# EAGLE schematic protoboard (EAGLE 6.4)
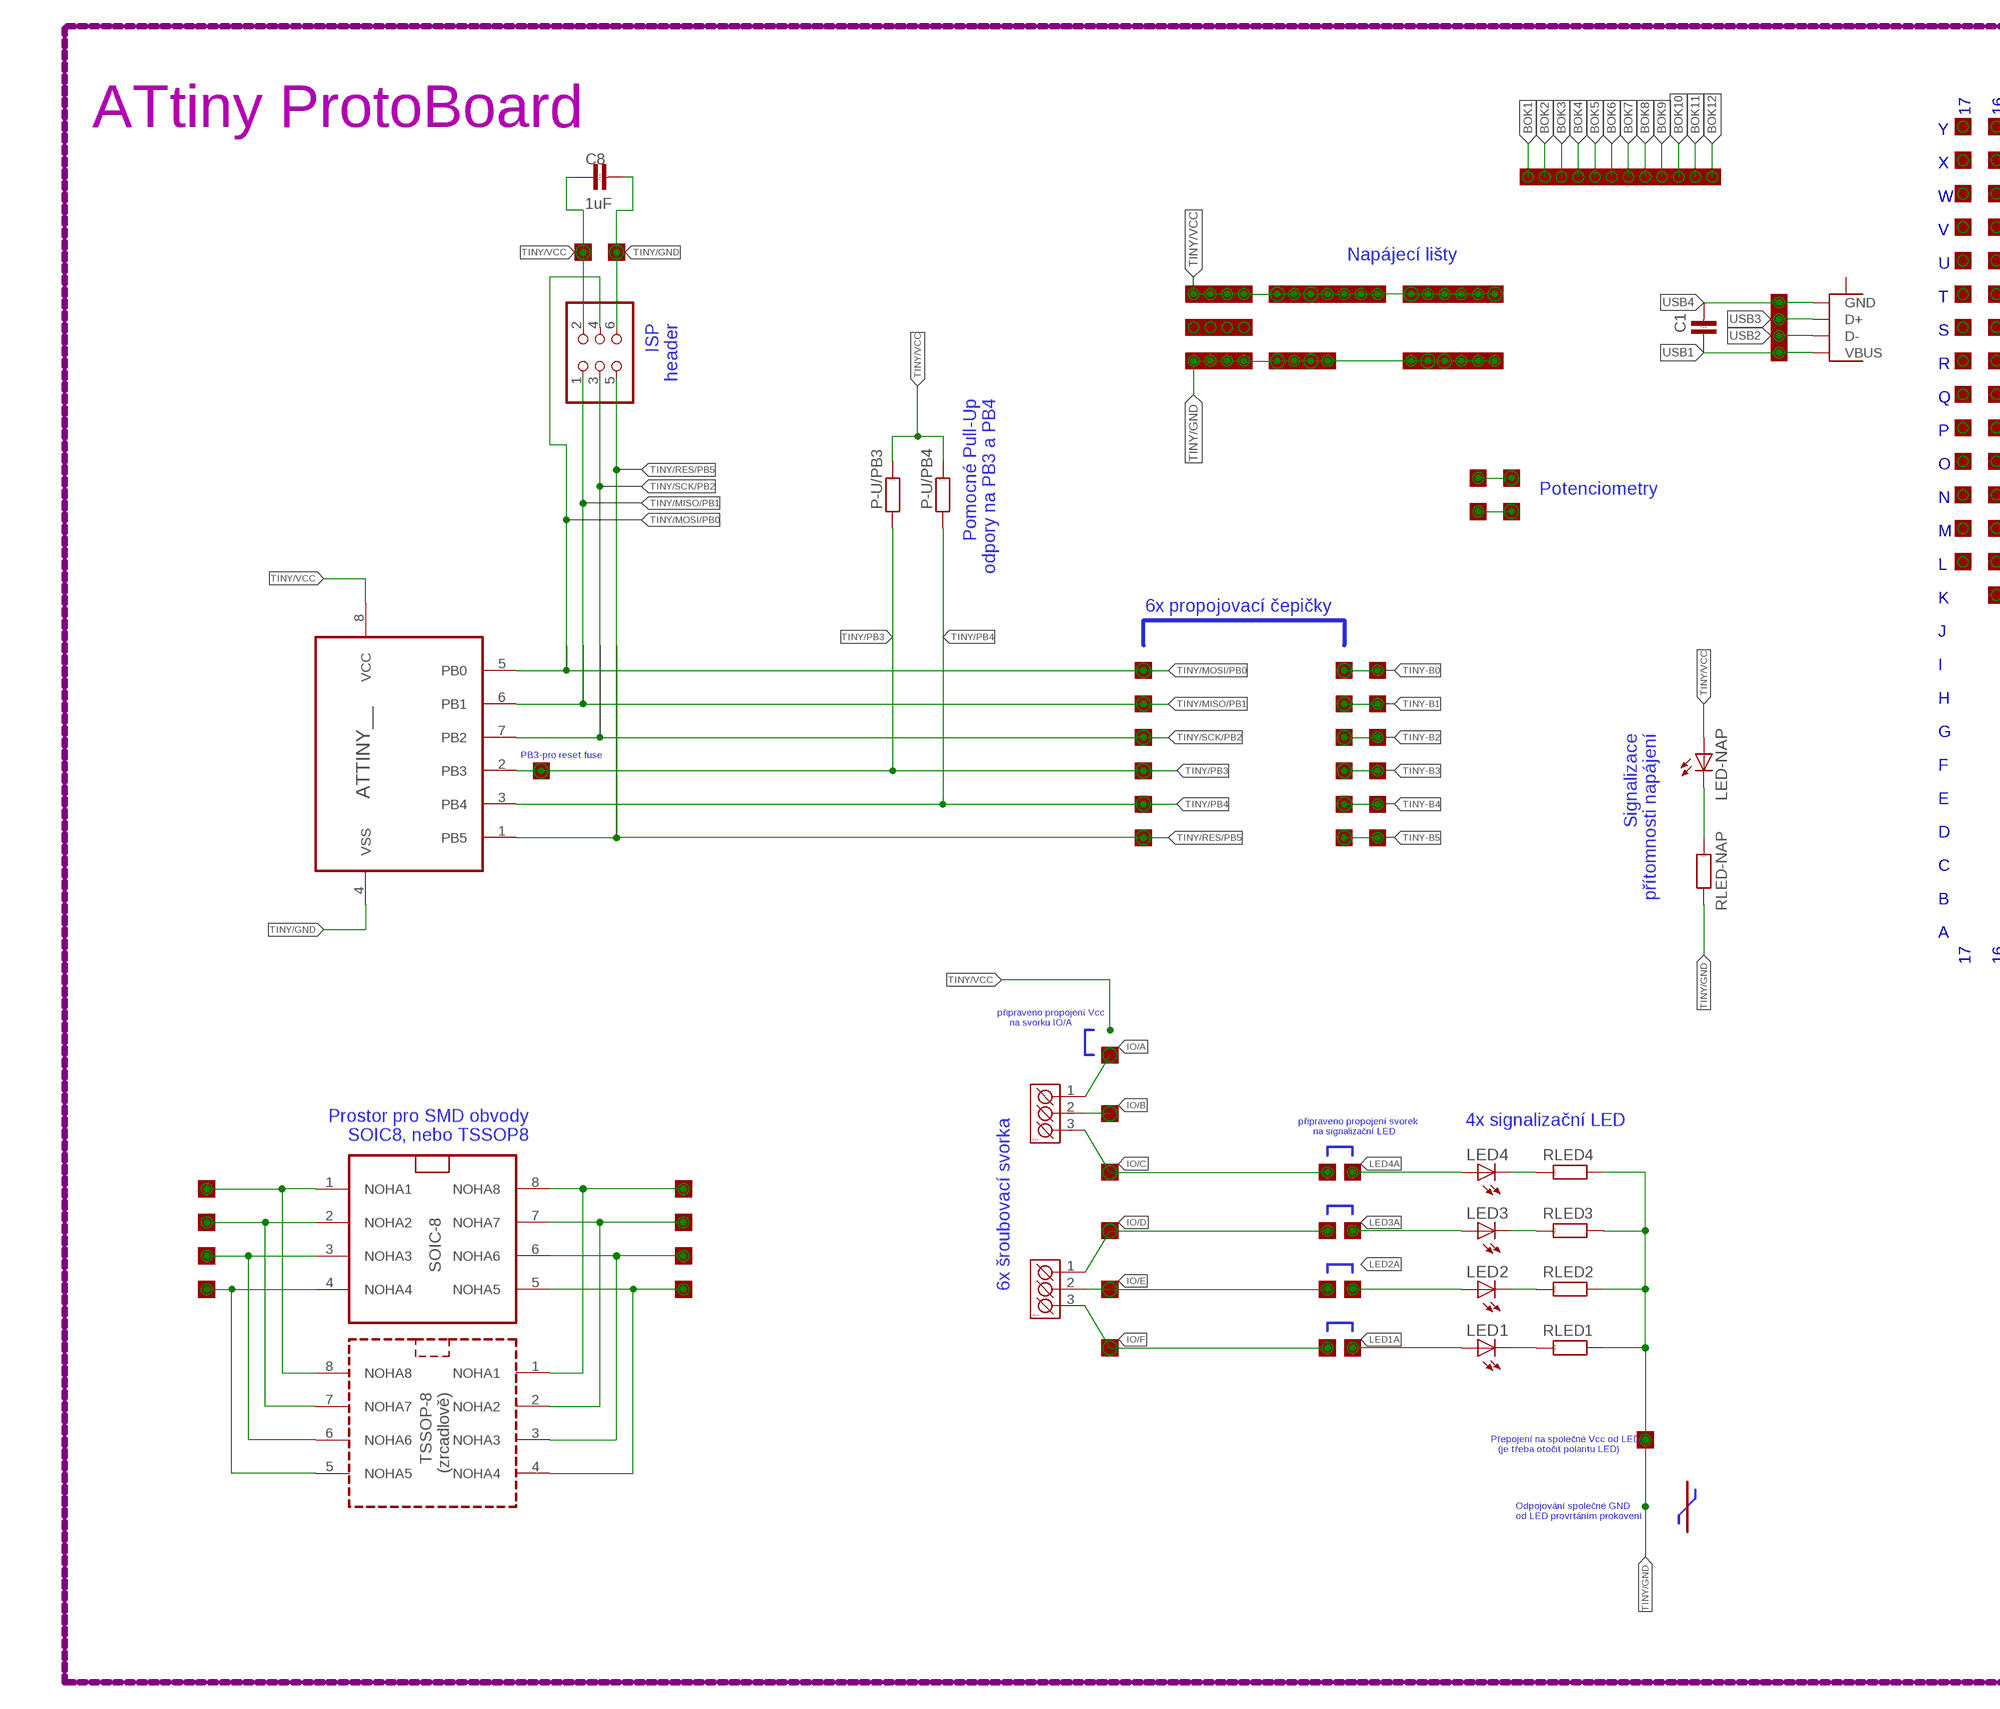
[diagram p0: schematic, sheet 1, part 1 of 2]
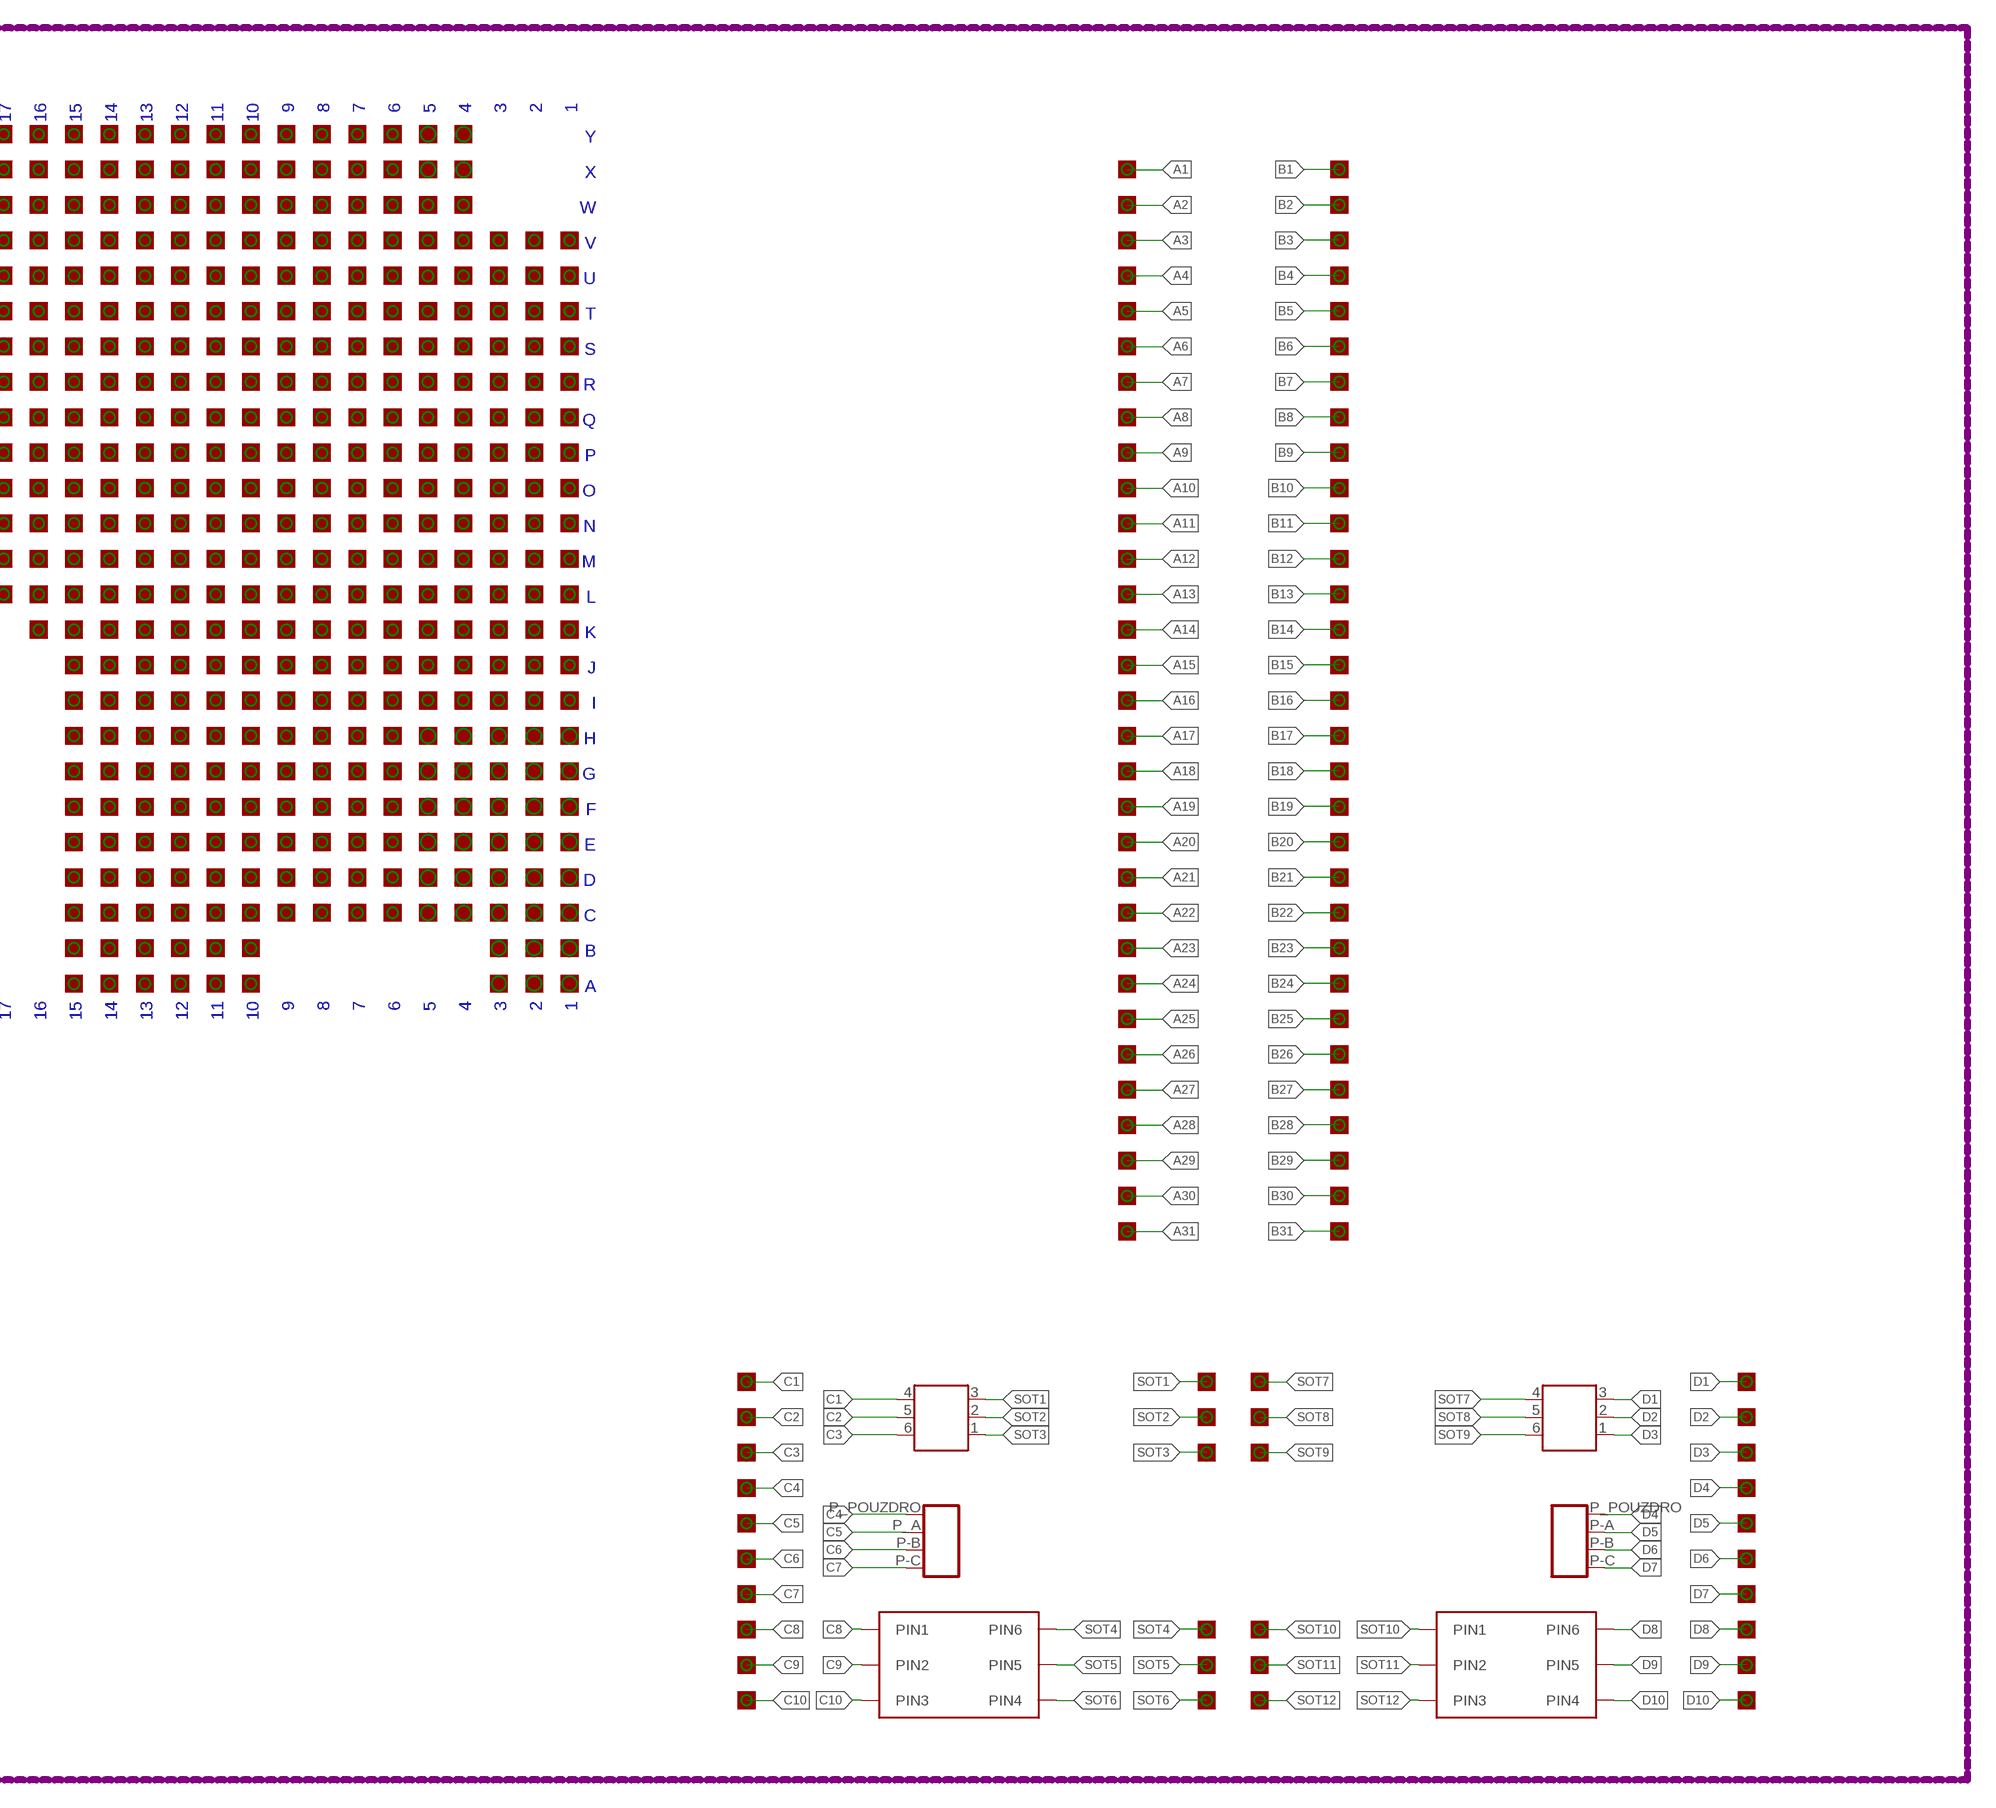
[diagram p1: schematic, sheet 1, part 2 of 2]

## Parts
ARK-A  PINHD-1X1  [1X01]
ARK-B  PINHD-1X1  [1X01]
ARK-C  PINHD-1X1  [1X01]
ARK-D  PINHD-1X1  [1X01]
ARK-E  PINHD-1X1  [1X01]
ARK-F  PINHD-1X1  [1X01]
ATTINY  ATTINY__  ATTINY13  [SOIC127P600X175-8N]
C1  C-KERAMIK_SMD_0805  [0805]
C8  1uF  C-KERAMIK_SMD_0805  [0805]
EMPTY1  SOIC-NIC  [SOIC127P600X175-8N]
EMPTY2  TSSOP-NIC  [TSSOP8]
IC1  AD8519KS  [SC70-5]
IC2  AD8519RJ  [SOT23-5]
J-A1  PINHD-1X1  [1X01]
J-A2  PINHD-1X1  [1X01]
J-A3  PINHD-1X1  [1X01]
J-A10  PINHD-1X1  [1X01]
J-A11  PINHD-1X1  [1X01]
J-A12  PINHD-1X1  [1X01]
J-A13  PINHD-1X1  [1X01]
J-A14  PINHD-1X1  [1X01]
J-A15  PINHD-1X1  [1X01]
J-B1  PINHD-1X1  [1X01]
J-B2  PINHD-1X1  [1X01]
J-B3  PINHD-1X1  [1X01]
J-B4  PINHD-1X1  [1X01]
J-B5  PINHD-1X1  [1X01]
J-B6  PINHD-1X1  [1X01]
J-B7  PINHD-1X1  [1X01]
J-B8  PINHD-1X1  [1X01]
J-B9  PINHD-1X1  [1X01]
J-B10  PINHD-1X1  [1X01]
J-B11  PINHD-1X1  [1X01]
J-B12  PINHD-1X1  [1X01]
J-B13  PINHD-1X1  [1X01]
J-B14  PINHD-1X1  [1X01]
J-B15  PINHD-1X1  [1X01]
J-C1  PINHD-1X1  [1X01]
J-C2  PINHD-1X1  [1X01]
J-C3  PINHD-1X1  [1X01]
J-C4  PINHD-1X1  [1X01]
J-C5  PINHD-1X1  [1X01]
J-C6  PINHD-1X1  [1X01]
J-C7  PINHD-1X1  [1X01]
J-C8  PINHD-1X1  [1X01]
J-C9  PINHD-1X1  [1X01]
J-C10  PINHD-1X1  [1X01]
J-C11  PINHD-1X1  [1X01]
J-C12  PINHD-1X1  [1X01]
J-C13  PINHD-1X1  [1X01]
J-C14  PINHD-1X1  [1X01]
J-C15  PINHD-1X1  [1X01]
J-D1  PINHD-1X1  [1X01]
J-D2  PINHD-1X1  [1X01]
J-D3  PINHD-1X1  [1X01]
J-D4  PINHD-1X1  [1X01]
J-D5  PINHD-1X1  [1X01]
J-D6  PINHD-1X1  [1X01]
J-D7  PINHD-1X1  [1X01]
J-D8  PINHD-1X1  [1X01]
J-D9  PINHD-1X1  [1X01]
J-D10  PINHD-1X1  [1X01]
J-D11  PINHD-1X1  [1X01]
J-D12  PINHD-1X1  [1X01]
J-D13  PINHD-1X1  [1X01]
J-D14  PINHD-1X1  [1X01]
J-D15  PINHD-1X1  [1X01]
J-E1  PINHD-1X1  [1X01]
J-E2  PINHD-1X1  [1X01]
J-E3  PINHD-1X1  [1X01]
J-E4  PINHD-1X1  [1X01]
J-E5  PINHD-1X1  [1X01]
J-E6  PINHD-1X1  [1X01]
J-E7  PINHD-1X1  [1X01]
J-E8  PINHD-1X1  [1X01]
J-E9  PINHD-1X1  [1X01]
J-E10  PINHD-1X1  [1X01]
J-E11  PINHD-1X1  [1X01]
J-E12  PINHD-1X1  [1X01]
J-E13  PINHD-1X1  [1X01]
J-E14  PINHD-1X1  [1X01]
J-E15  PINHD-1X1  [1X01]
J-F1  PINHD-1X1  [1X01]
J-F2  PINHD-1X1  [1X01]
J-F3  PINHD-1X1  [1X01]
J-F4  PINHD-1X1  [1X01]
J-F5  PINHD-1X1  [1X01]
J-F6  PINHD-1X1  [1X01]
J-F7  PINHD-1X1  [1X01]
J-F8  PINHD-1X1  [1X01]
J-F9  PINHD-1X1  [1X01]
J-F10  PINHD-1X1  [1X01]
J-F11  PINHD-1X1  [1X01]
J-F12  PINHD-1X1  [1X01]
J-F13  PINHD-1X1  [1X01]
J-F14  PINHD-1X1  [1X01]
J-F15  PINHD-1X1  [1X01]
J-G1  PINHD-1X1  [1X01]
J-G2  PINHD-1X1  [1X01]
J-G3  PINHD-1X1  [1X01]
J-G4  PINHD-1X1  [1X01]
J-G5  PINHD-1X1  [1X01]
J-G6  PINHD-1X1  [1X01]
J-G7  PINHD-1X1  [1X01]
J-G8  PINHD-1X1  [1X01]
J-G9  PINHD-1X1  [1X01]
J-G10  PINHD-1X1  [1X01]
J-G11  PINHD-1X1  [1X01]
J-G12  PINHD-1X1  [1X01]
J-G13  PINHD-1X1  [1X01]
J-G14  PINHD-1X1  [1X01]
J-G15  PINHD-1X1  [1X01]
J-H1  PINHD-1X1  [1X01]
J-H2  PINHD-1X1  [1X01]
J-H3  PINHD-1X1  [1X01]
J-H4  PINHD-1X1  [1X01]
J-H5  PINHD-1X1  [1X01]
J-H6  PINHD-1X1  [1X01]
J-H7  PINHD-1X1  [1X01]
J-H8  PINHD-1X1  [1X01]
J-H9  PINHD-1X1  [1X01]
J-H10  PINHD-1X1  [1X01]
J-H11  PINHD-1X1  [1X01]
J-H12  PINHD-1X1  [1X01]
J-H13  PINHD-1X1  [1X01]
J-H14  PINHD-1X1  [1X01]
J-H15  PINHD-1X1  [1X01]
J-HL-1  PINHD-1X1  [1X01]
J-HL-2  PINHD-1X1  [1X01]
J-HL-3  PINHD-1X1  [1X01]
J-HL-4  PINHD-1X1  [1X01]
J-I1  PINHD-1X1  [1X01]
J-I2  PINHD-1X1  [1X01]
J-I3  PINHD-1X1  [1X01]
J-I4  PINHD-1X1  [1X01]
J-I5  PINHD-1X1  [1X01]
J-I6  PINHD-1X1  [1X01]
J-I7  PINHD-1X1  [1X01]
J-I8  PINHD-1X1  [1X01]
J-I9  PINHD-1X1  [1X01]
J-I10  PINHD-1X1  [1X01]
J-I11  PINHD-1X1  [1X01]
J-I12  PINHD-1X1  [1X01]
J-I13  PINHD-1X1  [1X01]
J-I14  PINHD-1X1  [1X01]
J-I15  PINHD-1X1  [1X01]
J-J1  PINHD-1X1  [1X01]
J-J2  PINHD-1X1  [1X01]
J-J3  PINHD-1X1  [1X01]
J-J4  PINHD-1X1  [1X01]
J-J5  PINHD-1X1  [1X01]
J-J6  PINHD-1X1  [1X01]
J-J7  PINHD-1X1  [1X01]
J-J8  PINHD-1X1  [1X01]
J-J9  PINHD-1X1  [1X01]
J-J10  PINHD-1X1  [1X01]
J-J11  PINHD-1X1  [1X01]
J-J12  PINHD-1X1  [1X01]
J-J13  PINHD-1X1  [1X01]
J-J14  PINHD-1X1  [1X01]
J-J15  PINHD-1X1  [1X01]
J-K1  PINHD-1X1  [1X01]
J-K2  PINHD-1X1  [1X01]
J-K3  PINHD-1X1  [1X01]
J-K4  PINHD-1X1  [1X01]
J-K5  PINHD-1X1  [1X01]
J-K6  PINHD-1X1  [1X01]
J-K7  PINHD-1X1  [1X01]
J-K8  PINHD-1X1  [1X01]
J-K9  PINHD-1X1  [1X01]
J-K10  PINHD-1X1  [1X01]
J-K11  PINHD-1X1  [1X01]
J-K12  PINHD-1X1  [1X01]
J-K13  PINHD-1X1  [1X01]
J-K14  PINHD-1X1  [1X01]
J-K15  PINHD-1X1  [1X01]
J-K16  PINHD-1X1  [1X01]
J-L1  PINHD-1X1  [1X01]
J-L2  PINHD-1X1  [1X01]
J-L3  PINHD-1X1  [1X01]
J-L4  PINHD-1X1  [1X01]
J-L5  PINHD-1X1  [1X01]
J-L6  PINHD-1X1  [1X01]
J-L7  PINHD-1X1  [1X01]
J-L8  PINHD-1X1  [1X01]
J-L9  PINHD-1X1  [1X01]
J-L10  PINHD-1X1  [1X01]
J-L11  PINHD-1X1  [1X01]
J-L12  PINHD-1X1  [1X01]
J-L13  PINHD-1X1  [1X01]
J-L14  PINHD-1X1  [1X01]
J-L15  PINHD-1X1  [1X01]
J-L16  PINHD-1X1  [1X01]
J-L17  PINHD-1X1  [1X01]
J-LED1A  PINHD-1X1  [1X01]
J-LED1B  PINHD-1X1  [1X01]
J-LED2A  PINHD-1X1  [1X01]
J-LED2B  PINHD-1X1  [1X01]
J-LED3A  PINHD-1X1  [1X01]
J-LED3B  PINHD-1X1  [1X01]
J-LED4A  PINHD-1X1  [1X01]
J-LED4B  PINHD-1X1  [1X01]
J-M1  PINHD-1X1  [1X01]
J-M2  PINHD-1X1  [1X01]
J-M3  PINHD-1X1  [1X01]
J-M4  PINHD-1X1  [1X01]
J-M5  PINHD-1X1  [1X01]
J-M6  PINHD-1X1  [1X01]
J-M7  PINHD-1X1  [1X01]
J-M8  PINHD-1X1  [1X01]
J-M9  PINHD-1X1  [1X01]
J-M10  PINHD-1X1  [1X01]
J-M11  PINHD-1X1  [1X01]
J-M12  PINHD-1X1  [1X01]
J-M13  PINHD-1X1  [1X01]
J-M14  PINHD-1X1  [1X01]
J-M15  PINHD-1X1  [1X01]
J-M16  PINHD-1X1  [1X01]
J-M17  PINHD-1X1  [1X01]
J-N1  PINHD-1X1  [1X01]
J-N2  PINHD-1X1  [1X01]
J-N3  PINHD-1X1  [1X01]
J-N4  PINHD-1X1  [1X01]
J-N5  PINHD-1X1  [1X01]
J-N6  PINHD-1X1  [1X01]
J-N7  PINHD-1X1  [1X01]
J-N8  PINHD-1X1  [1X01]
J-N9  PINHD-1X1  [1X01]
J-N10  PINHD-1X1  [1X01]
J-N11  PINHD-1X1  [1X01]
J-N12  PINHD-1X1  [1X01]
J-N13  PINHD-1X1  [1X01]
J-N14  PINHD-1X1  [1X01]
J-N15  PINHD-1X1  [1X01]
J-N16  PINHD-1X1  [1X01]
J-N17  PINHD-1X1  [1X01]
J-O1  PINHD-1X1  [1X01]
J-O2  PINHD-1X1  [1X01]
J-O3  PINHD-1X1  [1X01]
J-O4  PINHD-1X1  [1X01]
J-O5  PINHD-1X1  [1X01]
J-O6  PINHD-1X1  [1X01]
J-O7  PINHD-1X1  [1X01]
J-O8  PINHD-1X1  [1X01]
J-O9  PINHD-1X1  [1X01]
J-O10  PINHD-1X1  [1X01]
J-O11  PINHD-1X1  [1X01]
J-O12  PINHD-1X1  [1X01]
J-O13  PINHD-1X1  [1X01]
J-O14  PINHD-1X1  [1X01]
J-O15  PINHD-1X1  [1X01]
J-O16  PINHD-1X1  [1X01]
J-O17  PINHD-1X1  [1X01]
J-P1  PINHD-1X1  [1X01]
J-P2  PINHD-1X1  [1X01]
J-P3  PINHD-1X1  [1X01]
J-P4  PINHD-1X1  [1X01]
J-P5  PINHD-1X1  [1X01]
J-P6  PINHD-1X1  [1X01]
J-P7  PINHD-1X1  [1X01]
J-P8  PINHD-1X1  [1X01]
J-P9  PINHD-1X1  [1X01]
J-P10  PINHD-1X1  [1X01]
J-P11  PINHD-1X1  [1X01]
J-P12  PINHD-1X1  [1X01]
J-P13  PINHD-1X1  [1X01]
J-P14  PINHD-1X1  [1X01]
J-P15  PINHD-1X1  [1X01]
J-P16  PINHD-1X1  [1X01]
J-P17  PINHD-1X1  [1X01]
J-Q1  PINHD-1X1  [1X01]
J-Q2  PINHD-1X1  [1X01]
J-Q3  PINHD-1X1  [1X01]
J-Q4  PINHD-1X1  [1X01]
J-Q5  PINHD-1X1  [1X01]
J-Q6  PINHD-1X1  [1X01]
J-Q7  PINHD-1X1  [1X01]
J-Q8  PINHD-1X1  [1X01]
J-Q9  PINHD-1X1  [1X01]
J-Q10  PINHD-1X1  [1X01]
J-Q11  PINHD-1X1  [1X01]
J-Q12  PINHD-1X1  [1X01]
J-Q13  PINHD-1X1  [1X01]
J-Q14  PINHD-1X1  [1X01]
J-Q15  PINHD-1X1  [1X01]
J-Q16  PINHD-1X1  [1X01]
J-Q17  PINHD-1X1  [1X01]
J-R1  PINHD-1X1  [1X01]
J-R2  PINHD-1X1  [1X01]
J-R3  PINHD-1X1  [1X01]
J-R4  PINHD-1X1  [1X01]
J-R5  PINHD-1X1  [1X01]
J-R6  PINHD-1X1  [1X01]
J-R7  PINHD-1X1  [1X01]
J-R8  PINHD-1X1  [1X01]
J-R9  PINHD-1X1  [1X01]
J-R10  PINHD-1X1  [1X01]
J-R11  PINHD-1X1  [1X01]
J-R12  PINHD-1X1  [1X01]
J-R13  PINHD-1X1  [1X01]
J-R14  PINHD-1X1  [1X01]
J-R15  PINHD-1X1  [1X01]
J-R16  PINHD-1X1  [1X01]
J-R17  PINHD-1X1  [1X01]
J-S1  PINHD-1X1  [1X01]
J-S2  PINHD-1X1  [1X01]
J-S3  PINHD-1X1  [1X01]
J-S4  PINHD-1X1  [1X01]
J-S5  PINHD-1X1  [1X01]
J-S6  PINHD-1X1  [1X01]
J-S7  PINHD-1X1  [1X01]
J-S8  PINHD-1X1  [1X01]
J-S9  PINHD-1X1  [1X01]
J-S10  PINHD-1X1  [1X01]
J-S11  PINHD-1X1  [1X01]
J-S12  PINHD-1X1  [1X01]
J-S13  PINHD-1X1  [1X01]
J-S14  PINHD-1X1  [1X01]
J-S15  PINHD-1X1  [1X01]
J-S16  PINHD-1X1  [1X01]
J-S17  PINHD-1X1  [1X01]
J-SOIC-1  PINHD-1X1  [1X01]
J-SOIC-2  PINHD-1X1  [1X01]
J-SOIC-3  PINHD-1X1  [1X01]
J-SOIC-4  PINHD-1X1  [1X01]
J-SOIC-6  PINHD-1X1  [1X01]
J-SOIC-7  PINHD-1X1  [1X01]
J-SOIC-8  PINHD-1X1  [1X01]
J-T1  PINHD-1X1  [1X01]
J-T2  PINHD-1X1  [1X01]
J-T3  PINHD-1X1  [1X01]
J-T4  PINHD-1X1  [1X01]
J-T5  PINHD-1X1  [1X01]
J-T6  PINHD-1X1  [1X01]
J-T7  PINHD-1X1  [1X01]
J-T8  PINHD-1X1  [1X01]
J-T9  PINHD-1X1  [1X01]
J-T10  PINHD-1X1  [1X01]
J-T11  PINHD-1X1  [1X01]
J-T12  PINHD-1X1  [1X01]
J-T13  PINHD-1X1  [1X01]
J-T14  PINHD-1X1  [1X01]
J-T15  PINHD-1X1  [1X01]
J-T16  PINHD-1X1  [1X01]
J-T17  PINHD-1X1  [1X01]
J-U1  PINHD-1X1  [1X01]
J-U2  PINHD-1X1  [1X01]
J-U3  PINHD-1X1  [1X01]
J-U4  PINHD-1X1  [1X01]
J-U5  PINHD-1X1  [1X01]
J-U6  PINHD-1X1  [1X01]
J-U7  PINHD-1X1  [1X01]
J-U8  PINHD-1X1  [1X01]
J-U9  PINHD-1X1  [1X01]
J-U10  PINHD-1X1  [1X01]
J-U11  PINHD-1X1  [1X01]
J-U12  PINHD-1X1  [1X01]
J-U13  PINHD-1X1  [1X01]
J-U14  PINHD-1X1  [1X01]
J-U15  PINHD-1X1  [1X01]
J-U16  PINHD-1X1  [1X01]
J-U17  PINHD-1X1  [1X01]
J-V1  PINHD-1X1  [1X01]
J-V2  PINHD-1X1  [1X01]
J-V3  PINHD-1X1  [1X01]
J-V4  PINHD-1X1  [1X01]
J-V5  PINHD-1X1  [1X01]
J-V6  PINHD-1X1  [1X01]
J-V7  PINHD-1X1  [1X01]
J-V8  PINHD-1X1  [1X01]
J-V9  PINHD-1X1  [1X01]
J-V10  PINHD-1X1  [1X01]
J-V11  PINHD-1X1  [1X01]
J-V12  PINHD-1X1  [1X01]
J-V13  PINHD-1X1  [1X01]
J-V14  PINHD-1X1  [1X01]
J-V15  PINHD-1X1  [1X01]
J-V16  PINHD-1X1  [1X01]
J-V17  PINHD-1X1  [1X01]
J-W4  PINHD-1X1  [1X01]
J-W5  PINHD-1X1  [1X01]
J-W6  PINHD-1X1  [1X01]
J-W7  PINHD-1X1  [1X01]
J-W8  PINHD-1X1  [1X01]
J-W9  PINHD-1X1  [1X01]
J-W10  PINHD-1X1  [1X01]
J-W11  PINHD-1X1  [1X01]
J-W12  PINHD-1X1  [1X01]
J-W13  PINHD-1X1  [1X01]
J-W14  PINHD-1X1  [1X01]
J-W15  PINHD-1X1  [1X01]
J-W16  PINHD-1X1  [1X01]
J-W17  PINHD-1X1  [1X01]
J-X4  PINHD-1X1  [1X01]
J-X5  PINHD-1X1  [1X01]
J-X6  PINHD-1X1  [1X01]
J-X7  PINHD-1X1  [1X01]
J-X8  PINHD-1X1  [1X01]
J-X9  PINHD-1X1  [1X01]
J-X10  PINHD-1X1  [1X01]
J-X11  PINHD-1X1  [1X01]
J-X12  PINHD-1X1  [1X01]
J-X13  PINHD-1X1  [1X01]
J-X14  PINHD-1X1  [1X01]
J-X15  PINHD-1X1  [1X01]
J-X16  PINHD-1X1  [1X01]
J-X17  PINHD-1X1  [1X01]
J-Y4  PINHD-1X1  [1X01]
J-Y5  PINHD-1X1  [1X01]
J-Y6  PINHD-1X1  [1X01]
J-Y7  PINHD-1X1  [1X01]
J-Y8  PINHD-1X1  [1X01]
J-Y9  PINHD-1X1  [1X01]
J-Y10  PINHD-1X1  [1X01]
J-Y11  PINHD-1X1  [1X01]
J-Y12  PINHD-1X1  [1X01]
J-Y13  PINHD-1X1  [1X01]
J-Y14  PINHD-1X1  [1X01]
J-Y15  PINHD-1X1  [1X01]
J-Y16  PINHD-1X1  [1X01]
J-Y17  PINHD-1X1  [1X01]
JP9  PINHD-1X1  [1X01]
JP19  PINHD-1X1  [1X01]
JP20  PINHD-1X1  [1X01]
JP21  PINHD-1X1  [1X01]
JP24  PINHD-1X1  [1X01]
JP25  PINHD-1X1  [1X01]
JP27  PINHD-1X1  [1X01]
JP28  PINHD-1X1  [1X01]
JP29  PINHD-1X1  [1X01]
JP30  PINHD-1X1  [1X01]
JP31  PINHD-1X1  [1X01]
JP32  PINHD-1X1  [1X01]
JP96  PINHD-1X1  [1X01]
JP117  PINHD-1X1  [1X01]
JP198  PINHD-1X1  [1X01]
K1  CZM_5/3  [CZM_5/3]
K2  CZM_5/3  [CZM_5/3]
LED1  L-HSMS-C650  [CHIPLED_1206]
LED2  L-HSMS-C650  [CHIPLED_1206]
LED3  L-HSMS-C650  [CHIPLED_1206]
LED4  L-HSMS-C650  [CHIPLED_1206]
LED-NAP  L-HSMY-C650  [CHIPLED_1206]
P-U/PB3  R_SMD_0805  [0805]
P-U/PB4  R_SMD_0805  [0805]
PIN1A  PINHD-1X1  [1X01]
PIN1B  PINHD-1X1  [1X01]
PIN1C  PINHD-1X1  [1X01]
PIN1D  PINHD-1X1  [1X01]
PIN2A  PINHD-1X1  [1X01]
PIN2B  PINHD-1X1  [1X01]
PIN2C  PINHD-1X1  [1X01]
PIN2D  PINHD-1X1  [1X01]
PIN3A  PINHD-1X1  [1X01]
PIN3B  PINHD-1X1  [1X01]
PIN3C  PINHD-1X1  [1X01]
PIN3D  PINHD-1X1  [1X01]
PIN4A  PINHD-1X1  [1X01]
PIN4B  PINHD-1X1  [1X01]
PIN4C  PINHD-1X1  [1X01]
PIN4D  PINHD-1X1  [1X01]
PIN5A  PINHD-1X1  [1X01]
PIN5B  PINHD-1X1  [1X01]
PIN5C  PINHD-1X1  [1X01]
PIN5D  PINHD-1X1  [1X01]
PIN6A  PINHD-1X1  [1X01]
PIN6B  PINHD-1X1  [1X01]
PIN6C  PINHD-1X1  [1X01]
PIN6D  PINHD-1X1  [1X01]
PIN7A  PINHD-1X1  [1X01]
PIN7B  PINHD-1X1  [1X01]
PIN7C  PINHD-1X1  [1X01]
PIN7D  PINHD-1X1  [1X01]
PIN8A  PINHD-1X1  [1X01]
PIN8B  PINHD-1X1  [1X01]
PIN8C  PINHD-1X1  [1X01]
PIN8D  PINHD-1X1  [1X01]
PIN9A  PINHD-1X1  [1X01]
PIN9B  PINHD-1X1  [1X01]
PIN9C  PINHD-1X1  [1X01]
PIN9D  PINHD-1X1  [1X01]
PIN10A  PINHD-1X1  [1X01]
PIN10B  PINHD-1X1  [1X01]
PIN10C  PINHD-1X1  [1X01]
PIN10D  PINHD-1X1  [1X01]
PIN11A  PINHD-1X1  [1X01]
PIN11B  PINHD-1X1  [1X01]
PIN12A  PINHD-1X1  [1X01]
PIN12B  PINHD-1X1  [1X01]
PIN13A  PINHD-1X1  [1X01]
PIN13B  PINHD-1X1  [1X01]
PIN14A  PINHD-1X1  [1X01]
PIN14B  PINHD-1X1  [1X01]
PIN15A  PINHD-1X1  [1X01]
PIN15B  PINHD-1X1  [1X01]
PIN16A  PINHD-1X1  [1X01]
PIN16B  PINHD-1X1  [1X01]
PIN17A  PINHD-1X1  [1X01]
PIN17B  PINHD-1X1  [1X01]
PIN18A  PINHD-1X1  [1X01]
PIN18B  PINHD-1X1  [1X01]
PIN19A  PINHD-1X1  [1X01]
PIN19B  PINHD-1X1  [1X01]
PIN20A  PINHD-1X1  [1X01]
PIN20B  PINHD-1X1  [1X01]
PIN21A  PINHD-1X1  [1X01]
PIN21B  PINHD-1X1  [1X01]
PIN22A  PINHD-1X1  [1X01]
PIN22B  PINHD-1X1  [1X01]
PIN23A  PINHD-1X1  [1X01]
PIN23B  PINHD-1X1  [1X01]
PIN24A  PINHD-1X1  [1X01]
PIN24B  PINHD-1X1  [1X01]
PIN25A  PINHD-1X1  [1X01]
PIN25B  PINHD-1X1  [1X01]
PIN26A  PINHD-1X1  [1X01]
PIN26B  PINHD-1X1  [1X01]
PIN27A  PINHD-1X1  [1X01]
PIN27B  PINHD-1X1  [1X01]
PIN28A  PINHD-1X1  [1X01]
PIN28B  PINHD-1X1  [1X01]
PIN29A  PINHD-1X1  [1X01]
PIN29B  PINHD-1X1  [1X01]
PIN30A  PINHD-1X1  [1X01]
PIN30B  PINHD-1X1  [1X01]
PIN31A  PINHD-1X1  [1X01]
PIN31B  PINHD-1X1  [1X01]
PIN-BOK1  PINHD-1X1  [1X01]
PIN-BOK2  PINHD-1X1  [1X01]
PIN-BOK3  PINHD-1X1  [1X01]
PIN-BOK4  PINHD-1X1  [1X01]
PIN-BOK5  PINHD-1X1  [1X01]
PIN-BOK6  PINHD-1X1  [1X01]
PIN-BOK7  PINHD-1X1  [1X01]
PIN-BOK8  PINHD-1X1  [1X01]
PIN-BOK9  PINHD-1X1  [1X01]
PIN-BOK10  PINHD-1X1  [1X01]
PIN-BOK11  PINHD-1X1  [1X01]
PIN-BOK12  PINHD-1X1  [1X01]
PIN-SOT1  PINHD-1X1  [1X01]
PIN-SOT2  PINHD-1X1  [1X01]
PIN-SOT3  PINHD-1X1  [1X01]
PIN-SOT4  PINHD-1X1  [1X01]
PIN-SOT5  PINHD-1X1  [1X01]
PIN-SOT6  PINHD-1X1  [1X01]
PIN-SOT7  PINHD-1X1  [1X01]
PIN-SOT8  PINHD-1X1  [1X01]
PIN-SOT9  PINHD-1X1  [1X01]
PIN-SOT10  PINHD-1X1  [1X01]
PIN-SOT11  PINHD-1X1  [1X01]
PIN-SOT12  PINHD-1X1  [1X01]
PINGND-1  PINHD-1X1  [1X01]
PINGND-2  PINHD-1X1  [1X01]
PINGND-3  PINHD-1X1  [1X01]
PINGND-4  PINHD-1X1  [1X01]
PINGND-5  PINHD-1X1  [1X01]
PINGND-6  PINHD-1X1  [1X01]
PINGND-7  PINHD-1X1  [1X01]
PINGND-8  PINHD-1X1  [1X01]
PINGND-9  PINHD-1X1  [1X01]
PINGND-10  PINHD-1X1  [1X01]
PINGND-11  PINHD-1X1  [1X01]
PINGND-12  PINHD-1X1  [1X01]
PINGND-13  PINHD-1X1  [1X01]
PINGND-14  PINHD-1X1  [1X01]
PINPOT1A  PINHD-1X1  [1X01]
PINPOT1B  PINHD-1X1  [1X01]
PINPOT2A  PINHD-1X1  [1X01]
PINPOT2B  PINHD-1X1  [1X01]
PINUSB1  PINHD-1X1  [1X01]
PINUSB2  PINHD-1X1  [1X01]
PINUSB3  PINHD-1X1  [1X01]
PINUSB4  PINHD-1X1  [1X01]
PINVCC-1  PINHD-1X1  [1X01]
PINVCC-2  PINHD-1X1  [1X01]
PINVCC-3  PINHD-1X1  [1X01]
PINVCC-4  PINHD-1X1  [1X01]
PINVCC-5  PINHD-1X1  [1X01]
PINVCC-6  PINHD-1X1  [1X01]
PINVCC-7  PINHD-1X1  [1X01]
PINVCC-8  PINHD-1X1  [1X01]
PINVCC-9  PINHD-1X1  [1X01]
PINVCC-10  PINHD-1X1  [1X01]
PINVCC-11  PINHD-1X1  [1X01]
PINVCC-12  PINHD-1X1  [1X01]
PINVCC-13  PINHD-1X1  [1X01]
PINVCC-14  PINHD-1X1  [1X01]
PINVCC-15  PINHD-1X1  [1X01]
PINVCC-16  PINHD-1X1  [1X01]
PINVCC-17  PINHD-1X1  [1X01]
PINVCC-18  PINHD-1X1  [1X01]
RLED1  R_SMD_0805  [0805]
RLED2  R_SMD_0805  [0805]
RLED3  R_SMD_0805  [0805]
RLED4  R_SMD_0805  [0805]
RLED-NAP  R_SMD_0805  [0805]
SOIC-5  PINHD-1X1  [1X01]
TINY-ISP  PINHD-2X3  [2X03]
U1  WS2812  WS2812"  [LED-TRICOLOR-5050-IC]
U2  WS2812  WS2812"  [LED-TRICOLOR-5050-IC]
U6  V_REG_78XX  [SOT223]
U7  +12v  V_REG_78XX7812  [TO-252]
X1  USBPTH  [USB-B-PTH]

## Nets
A1: PIN1A.1
A2: PIN2A.1
A3: PIN3A.1
A4: PIN4A.1
A5: PIN5A.1
A6: PIN6A.1
A7: PIN7A.1
A8: PIN8A.1
A9: PIN9A.1
A10: PIN10A.1
A11: PIN11A.1
A12: PIN12A.1
A13: PIN13A.1
A14: PIN14A.1
A15: PIN15A.1
A16: PIN16A.1
A17: PIN17A.1
A18: PIN18A.1
A19: PIN19A.1
A20: PIN20A.1
A21: PIN21A.1
A22: PIN22A.1
A23: PIN23A.1
A24: PIN24A.1
A25: PIN25A.1
A26: PIN26A.1
A27: PIN27A.1
A28: PIN28A.1
A29: PIN29A.1
A30: PIN30A.1
A31: PIN31A.1
B1: PIN1B.1
B2: PIN2B.1
B3: PIN3B.1
B4: PIN4B.1
B5: PIN5B.1
B6: PIN6B.1
B7: PIN7B.1
B8: PIN8B.1
B9: PIN9B.1
B10: PIN10B.1
B11: PIN11B.1
B12: PIN12B.1
B13: PIN13B.1
B14: PIN14B.1
B15: PIN15B.1
B16: PIN16B.1
B17: PIN17B.1
B18: PIN18B.1
B19: PIN19B.1
B20: PIN20B.1
B21: PIN21B.1
B22: PIN22B.1
B23: PIN23B.1
B24: PIN24B.1
B25: PIN25B.1
B26: PIN26B.1
B27: PIN27B.1
B28: PIN28B.1
B29: PIN29B.1
B30: PIN30B.1
B31: PIN31B.1
BOK1: PIN-BOK1.1
BOK2: PIN-BOK2.1
BOK3: PIN-BOK3.1
BOK4: PIN-BOK4.1
BOK5: PIN-BOK5.1
BOK6: PIN-BOK6.1
BOK7: PIN-BOK7.1
BOK8: PIN-BOK8.1
BOK9: PIN-BOK9.1
BOK10: PIN-BOK10.1
BOK11: PIN-BOK11.1
BOK12: PIN-BOK12.1
C1: IC2.4(PIN4) PIN1C.1
C2: IC2.5(PIN5) PIN2C.1
C3: IC2.6(PIN6) PIN3C.1
C4: PIN4C.1 U6.P_POUZDRO(IN)
C5: PIN5C.1 U6.P_A(GND)
C6: PIN6C.1 U6.P-B(OUT)
C7: PIN7C.1 U6.P-C(PIN1)
C8: PIN8C.1 U1.1(PIN1)
C9: PIN9C.1 U1.2(PIN2)
C10: PIN10C.1 U1.3(PIN3)
D1: IC1.3(PIN3) PIN1D.1
D2: IC1.2(PIN2) PIN2D.1
D3: IC1.1(PIN1) PIN3D.1
D4: PIN4D.1 U7.P_POUZDRO(PIN1)
D5: PIN5D.1 U7.P-A(OUT)
D6: PIN6D.1 U7.P-B(GND)
D7: PIN7D.1 U7.P-C(IN)
D8: PIN8D.1 U2.6(PIN6)
D9: PIN9D.1 U2.5(PIN5)
D10: PIN10D.1 U2.4(PIN4)
IO/A: ARK-A.1 K1.1(K1)
IO/B: ARK-B.1 K1.2(K2)
IO/C: ARK-C.1 J-LED1A.1 K1.3(K3)
IO/D: ARK-D.1 J-LED2A.1 K2.1(K1)
IO/E: ARK-E.1 J-LED3A.1 K2.2(K2)
IO/F: ARK-F.1 J-LED4A.1 K2.3(K3)
LED1A: J-LED1B.1 LED1.A
LED2A: J-LED2B.1 LED2.A
LED3A: J-LED3B.1 LED3.A
LED4A: J-LED4B.1 LED4.A
LEDK1: LED1.C RLED1.2
LEDK2: LED2.C RLED2.2
LEDK3: LED3.C RLED3.2
LEDK4: LED4.C RLED4.2
LEDNAP-K: LED-NAP.C RLED-NAP.2
POT1: PINPOT1A.1 PINPOT1B.1
POT2: PINPOT2A.1 PINPOT2B.1
SOT1: IC2.3(PIN3) PIN-SOT1.1
SOT2: IC2.2(PIN2) PIN-SOT2.1
SOT3: IC2.1(PIN1) PIN-SOT3.1
SOT4: PIN-SOT4.1 U1.6(PIN6)
SOT5: PIN-SOT5.1 U1.5(PIN5)
SOT6: PIN-SOT6.1 U1.4(PIN4)
SOT7: IC1.4(PIN4) PIN-SOT7.1
SOT8: IC1.5(PIN5) PIN-SOT8.1
SOT9: IC1.6(PIN6) PIN-SOT9.1
SOT10: PIN-SOT10.1 U2.1(PIN1)
SOT11: PIN-SOT11.1 U2.2(PIN2)
SOT12: PIN-SOT12.1 U2.3(PIN3)
TINY-B0: J-B4.1 JP24.1
TINY-B1: J-B5.1 JP21.1
TINY-B2: J-B6.1 JP20.1
TINY-B3: J-B9.1 JP9.1
TINY-B4: J-B8.1 JP25.1
TINY-B5: J-B7.1 JP19.1
TINY/GND: ATTINY.4(VSS) C8.2 JP117.1 JP198.1 PINGND-1.1 PINGND-2.1 PINGND-3.1 PINGND-4.1 PINGND-5.1 PINGND-6.1 PINGND-7.1 PINGND-8.1 PINGND-9.1 PINGND-10.1 PINGND-11.1 PINGND-12.1 PINGND-13.1 PINGND-14.1 RLED1.1 RLED2.1 RLED3.1 RLED4.1 RLED-NAP.1 TINY-ISP.6
TINY/MISO/PB1: ATTINY.6(PB1) JP28.1 TINY-ISP.1
TINY/MOSI/PB0: ATTINY.5(PB0) JP27.1 TINY-ISP.4
TINY/PB3: ATTINY.2(PB3) JP31.1 JP96.1 P-U/PB3.1
TINY/PB4: ATTINY.3(PB4) JP32.1 P-U/PB4.1
TINY/RES/PB5: ATTINY.1(PB5) JP30.1 TINY-ISP.5
TINY/SCK/PB2: ATTINY.7(PB2) JP29.1 TINY-ISP.3
TINY/SOIC1: EMPTY1.1(NOHA1) EMPTY2.8(NOHA8) J-SOIC-1.1
TINY/SOIC2: EMPTY1.2(NOHA2) EMPTY2.7(NOHA7) J-SOIC-2.1
TINY/SOIC3: EMPTY1.3(NOHA3) EMPTY2.6(NOHA6) J-SOIC-3.1
TINY/SOIC4: EMPTY1.4(NOHA4) EMPTY2.5(NOHA5) J-SOIC-4.1
TINY/SOIC5: EMPTY1.5(NOHA5) EMPTY2.4(NOHA4) SOIC-5.1
TINY/SOIC6: EMPTY1.6(NOHA6) EMPTY2.3(NOHA3) J-SOIC-6.1
TINY/SOIC7: EMPTY1.7(NOHA7) EMPTY2.2(NOHA2) J-SOIC-7.1
TINY/SOIC8: EMPTY1.8(NOHA8) EMPTY2.1(NOHA1) J-SOIC-8.1
TINY/VCC: ATTINY.8(VCC) C8.1 LED-NAP.A P-U/PB3.2 P-U/PB4.2 PINVCC-1.1 PINVCC-2.1 PINVCC-3.1 PINVCC-4.1 PINVCC-5.1 PINVCC-6.1 PINVCC-7.1 PINVCC-8.1 PINVCC-9.1 PINVCC-10.1 PINVCC-11.1 PINVCC-12.1 PINVCC-13.1 PINVCC-14.1 PINVCC-15.1 PINVCC-16.1 PINVCC-17.1 PINVCC-18.1 TINY-ISP.2
USB1: C1.1 PINUSB1.1 X1.VBUS
USB2: PINUSB2.1 X1.D-
USB3: PINUSB3.1 X1.D+
USB4: C1.2 PINUSB4.1 X1.GND
Unconnected: J-A1.1 J-A2.1 J-A3.1 J-A10.1 J-A11.1 J-A12.1 J-A13.1 J-A14.1 J-A15.1 J-B1.1 J-B2.1 J-B3.1 J-B10.1 J-B11.1 J-B12.1 J-B13.1 J-B14.1 J-B15.1 J-C1.1 J-C2.1 J-C3.1 J-C4.1 J-C5.1 J-C6.1 J-C7.1 J-C8.1 J-C9.1 J-C10.1 J-C11.1 J-C12.1 J-C13.1 J-C14.1 J-C15.1 J-D1.1 J-D2.1 J-D3.1 J-D4.1 J-D5.1 J-D6.1 J-D7.1 J-D8.1 J-D9.1 J-D10.1 J-D11.1 J-D12.1 J-D13.1 J-D14.1 J-D15.1 J-E1.1 J-E2.1 J-E3.1 J-E4.1 J-E5.1 J-E6.1 J-E7.1 J-E8.1 J-E9.1 J-E10.1 J-E11.1 J-E12.1 J-E13.1 J-E14.1 J-E15.1 J-F1.1 J-F2.1 J-F3.1 J-F4.1 J-F5.1 J-F6.1 J-F7.1 J-F8.1 J-F9.1 J-F10.1 J-F11.1 J-F12.1 J-F13.1 J-F14.1 J-F15.1 J-G1.1 J-G2.1 J-G3.1 J-G4.1 J-G5.1 J-G6.1 J-G7.1 J-G8.1 J-G9.1 J-G10.1 J-G11.1 J-G12.1 J-G13.1 J-G14.1 J-G15.1 J-H1.1 J-H2.1 J-H3.1 J-H4.1 J-H5.1 J-H6.1 J-H7.1 J-H8.1 J-H9.1 J-H10.1 J-H11.1 J-H12.1 J-H13.1 J-H14.1 J-H15.1 J-HL-1.1 J-HL-2.1 J-HL-3.1 J-HL-4.1 J-I1.1 J-I2.1 J-I3.1 J-I4.1 J-I5.1 J-I6.1 J-I7.1 J-I8.1 J-I9.1 J-I10.1 J-I11.1 J-I12.1 J-I13.1 J-I14.1 J-I15.1 J-J1.1 J-J2.1 J-J3.1 J-J4.1 J-J5.1 J-J6.1 J-J7.1 J-J8.1 J-J9.1 J-J10.1 J-J11.1 J-J12.1 J-J13.1 J-J14.1 J-J15.1 J-K1.1 J-K2.1 J-K3.1 J-K4.1 J-K5.1 J-K6.1 J-K7.1 J-K8.1 J-K9.1 J-K10.1 J-K11.1 J-K12.1 J-K13.1 J-K14.1 J-K15.1 J-K16.1 J-L1.1 J-L2.1 J-L3.1 J-L4.1 J-L5.1 J-L6.1 J-L7.1 J-L8.1 J-L9.1 J-L10.1 J-L11.1 J-L12.1 J-L13.1 J-L14.1 J-L15.1 J-L16.1 J-L17.1 J-M1.1 J-M2.1 J-M3.1 J-M4.1 J-M5.1 J-M6.1 J-M7.1 J-M8.1 J-M9.1 J-M10.1 J-M11.1 J-M12.1 J-M13.1 J-M14.1 J-M15.1 J-M16.1 J-M17.1 J-N1.1 J-N2.1 J-N3.1 J-N4.1 J-N5.1 J-N6.1 J-N7.1 J-N8.1 J-N9.1 J-N10.1 J-N11.1 J-N12.1 J-N13.1 J-N14.1 J-N15.1 J-N16.1 J-N17.1 J-O1.1 J-O2.1 J-O3.1 J-O4.1 J-O5.1 J-O6.1 J-O7.1 J-O8.1 J-O9.1 J-O10.1 J-O11.1 J-O12.1 J-O13.1 J-O14.1 J-O15.1 J-O16.1 J-O17.1 J-P1.1 J-P2.1 J-P3.1 J-P4.1 J-P5.1 J-P6.1 J-P7.1 J-P8.1 J-P9.1 J-P10.1 J-P11.1 J-P12.1 J-P13.1 J-P14.1 J-P15.1 J-P16.1 J-P17.1 J-Q1.1 J-Q2.1 J-Q3.1 J-Q4.1 J-Q5.1 J-Q6.1 J-Q7.1 J-Q8.1 J-Q9.1 J-Q10.1 J-Q11.1 J-Q12.1 J-Q13.1 J-Q14.1 J-Q15.1 J-Q16.1 J-Q17.1 J-R1.1 J-R2.1 J-R3.1 J-R4.1 J-R5.1 J-R6.1 J-R7.1 J-R8.1 J-R9.1 J-R10.1 J-R11.1 J-R12.1 J-R13.1 J-R14.1 J-R15.1 J-R16.1 J-R17.1 J-S1.1 J-S2.1 J-S3.1 J-S4.1 J-S5.1 J-S6.1 J-S7.1 J-S8.1 J-S9.1 J-S10.1 J-S11.1 J-S12.1 J-S13.1 J-S14.1 J-S15.1 J-S16.1 J-S17.1 J-T1.1 J-T2.1 J-T3.1 J-T4.1 J-T5.1 J-T6.1 J-T7.1 J-T8.1 J-T9.1 J-T10.1 J-T11.1 J-T12.1 J-T13.1 J-T14.1 J-T15.1 J-T16.1 J-T17.1 J-U1.1 J-U2.1 J-U3.1 J-U4.1 J-U5.1 J-U6.1 J-U7.1 J-U8.1 J-U9.1 J-U10.1 J-U11.1 J-U12.1 J-U13.1 J-U14.1 J-U15.1 J-U16.1 J-U17.1 J-V1.1 J-V2.1 J-V3.1 J-V4.1 J-V5.1 J-V6.1 J-V7.1 J-V8.1 J-V9.1 J-V10.1 J-V11.1 J-V12.1 J-V13.1 J-V14.1 J-V15.1 J-V16.1 J-V17.1 J-W4.1 J-W5.1 J-W6.1 J-W7.1 J-W8.1 J-W9.1 J-W10.1 J-W11.1 J-W12.1 J-W13.1 J-W14.1 J-W15.1 J-W16.1 J-W17.1 J-X4.1 J-X5.1 J-X6.1 J-X7.1 J-X8.1 J-X9.1 J-X10.1 J-X11.1 J-X12.1 J-X13.1 J-X14.1 J-X15.1 J-X16.1 J-X17.1 J-Y4.1 J-Y5.1 J-Y6.1 J-Y7.1 J-Y8.1 J-Y9.1 J-Y10.1 J-Y11.1 J-Y12.1 J-Y13.1 J-Y14.1 J-Y15.1 J-Y16.1 J-Y17.1 X1.P$2(SHIELD)

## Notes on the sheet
- ATtiny ProtoBoard
- 17 | 16 | 15 | 14 | 13 | 12 | 11 | 10 | 9 | 8 | 7 | 6 | 5 | 4 | 3 | 2 | 1
- Y | Y
- X | X
- W | W
- V | V
- Napájecí lišty
- U | U
- T | T
- ISP
  header
- S | S
- R | R
- Pomocné Pull-Up
  odpory na PB3 a PB4
- Q | Q
- P | P
- O | O
- Potenciometry
- N | N
- M | M
- L | L
- 6x propojovací čepičky | K | K
- J | J
- I | I
- H | H
- Signalizace
  přítomnosti napájení
- G | G
- PB3-pro reset fuse
- F | F
- E | E
- D | D
- C | C
- B | B
- A | A
- 17 | 16 | 15 | 14 | 13 | 12 | 11 | 10 | 9 | 8 | 7 | 6 | 5 | 4 | 3 | 2 | 1
- připraveno propojení Vcc
       na svorku IO/A
- Prostor pro SMD obvody
   SOIC8, nebo TSSOP8
- 6x šroubovací svorka
- 4x signalizační LED
- připraveno propojení svorek 
        na signalizační LED
- SOIC-8
- Přepojení na společné Vcc od LED
     (je třeba otočit polaritu LED)
- TSSOP-8
  (zrcadlově)
- Odpojování společné GND
  od LED provrtáním prokovení

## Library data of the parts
ARK-A ARK-B ARK-C ARK-D ARK-E ARK-F J-A1-J-A3 J-B1-J-B3 J-C1-J-C5 J-D1-J-D5 J-E1-J-E5 J-F1-J-F5 J-G1-J-G5 J-H1-J-H5 J-X4 J-X5 J-Y4 J-Y5 JP9 JP19-JP21 JP24 JP25 JP27-JP32 JP96 JP117 PINGND-5 PINGND-7 PINGND-10 PINGND-11 PINPOT1B PINPOT2B PINVCC-5 PINVCC-7 PINVCC-12 PINVCC-17 PINVCC-18 = jedenpin:PINHD-1X1: PIN HEADER
ATTINY = ATTiny13:ATTINY13: ATTINY13; PACKAGE: SOIC-8
C1 C8 = #PaJa_30:C-KERAMIK: Kondenzator - keramicky
EMPTY1 = soic-nic:SOIC-NIC: SOIC-NIC; PACKAGE: SOIC-8
EMPTY2 = tssop-nic:TSSOP-NIC: TSSOP-NIC; PACKAGE: TSSOP-8
IC1 = adpouzdra:AD8519: 8 MHz Rail-to-Rail Operational Amplifiers Source: http://www.analog.com/static/imported-files/data_sheets/AD8519_8529.pdf; OC_FARNELL: unknown; OC_NEWARK: unknown
IC2 = adpouzdra:AD8519: 8 MHz Rail-to-Rail Operational Amplifiers Source: http://www.analog.com/static/imported-files/data_sheets/AD8519_8529.pdf; MF: ALTERA CORPORATION; MPN: AD8519ARTZ-REEL7; OC_FARNELL: 1464960; OC_NEWARK: 59K6794
J-A10-J-A15 J-B4-J-B15 J-C6-J-C15 J-D6-J-D15 J-E6-J-E15 J-F6-J-F15 J-G6-J-G15 J-H6-J-H15 J-HL-1-J-HL-4 J-I1-J-I15 J-J1-J-J15 J-K1-J-K16 J-L1-J-L17 J-LED1A J-LED1B J-LED2A J-LED2B J-LED3A J-LED3B J-LED4A J-LED4B J-M1-J-M17 J-N1-J-N17 J-O1-J-O17 J-P1-J-P17 J-Q1-J-Q17 J-R1-J-R17 J-S1-J-S17 J-SOIC-1-J-SOIC-4 J-SOIC-6-J-SOIC-8 J-T1-J-T17 J-U1-J-U17 J-V1-J-V17 J-W4-J-W17 J-X6-J-X17 J-Y6-J-Y17 JP198 PIN1A PIN1B PIN1C PIN1D PIN2A PIN2B PIN2C PIN2D PIN3A PIN3B PIN3C PIN3D PIN4A PIN4B PIN4C PIN4D PIN5A PIN5B PIN5C PIN5D PIN6A PIN6B PIN6C PIN6D PIN7A PIN7B PIN7C PIN7D PIN8A PIN8B PIN8C PIN8D PIN9A PIN9B PIN9C PIN9D PIN10A PIN10B PIN10C PIN10D PIN11A PIN11B PIN12A PIN12B PIN13A PIN13B PIN14A PIN14B PIN15A PIN15B PIN16A PIN16B PIN17A PIN17B PIN18A PIN18B PIN19A PIN19B PIN20A PIN20B PIN21A PIN21B PIN22A PIN22B PIN23A PIN23B PIN24A PIN24B PIN25A PIN25B PIN26A PIN26B PIN27A PIN27B PIN28A PIN28B PIN29A PIN29B PIN30A PIN30B PIN31A PIN31B PIN-BOK1-PIN-BOK12 PIN-SOT1-PIN-SOT12 PINGND-1-PINGND-4 PINGND-6 PINGND-8 PINGND-9 PINGND-12-PINGND-14 PINPOT1A PINPOT2A PINUSB1-PINUSB4 PINVCC-1-PINVCC-4 PINVCC-6 PINVCC-8-PINVCC-11 PINVCC-13-PINVCC-16 SOIC-5 = obycpin:PINHD-1X1: PIN HEADER
K1 K2 = #PaJa_konektory:CZM_5/3: Svorkovnice - roztec 5,08mm - trojita 13,5A/250V
LED1-LED4 = LED diody:L-HSMS-C650: LED SMD
LED-NAP = LED diody:L-HSMY-C650: LED SMD
P-U/PB3 P-U/PB4 RLED1-RLED4 RLED-NAP = #PaJa_30:R: Rezistor
TINY-ISP = pinhead:PINHD-2X3: PIN HEADER
U1 U2 = ws2812:WS2812: Jen piny pr RGB LED; PROD_ID: DIO-11598
U6 = stabilizatory_pouzdra:V_REG_78XX: Voltage Regulator Standard 78xx regulator. IGO (Input Ground Output). Spark Fun Electronics SKU : COM-00107
U7 = stabilizatory_pouzdra:V_REG_78XX: Voltage Regulator Standard 78xx regulator. IGO (Input Ground Output). Spark Fun Electronics SKU : COM-00107; PROD_ID: VREG-12370
X1 = USB-B:USB: USB Connectors USB-B-PTH is fully proven SKU : PRT-00139 USB-miniB is fully proven SKU : PRT-00587 USB-A-PCB is untested. USB-A-H is C@H proven USB-B-SMT is throughly reviewed, but untested. Needs silkscreen touching up. USB-A-S has not been used/tested USB-MB-H has not been used/tested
